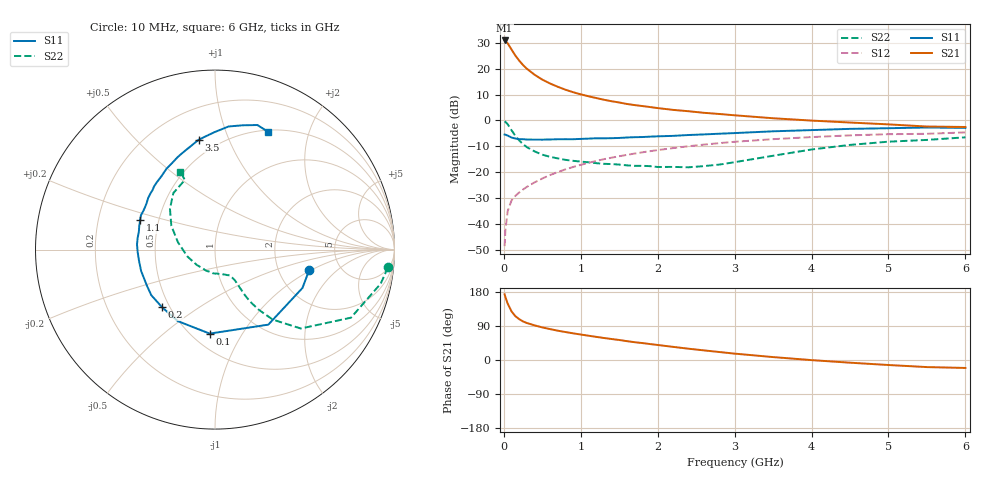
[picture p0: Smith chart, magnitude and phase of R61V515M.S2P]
! SIEMENS Small Signal Semiconductors
! BFR193
! Si NPN RF Bipolar Junction Transistor in SOT23
! VCE = 1.5 V  IC = 15 mA
! Common Emitter S-Parameters:  May  1996
# GHz  S  MA  R  50
!  f  S11  S21  S12  S22
! GHz  MAG  ANG  MAG  ANG  MAG  ANG  MAG  ANG
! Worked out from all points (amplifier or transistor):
!   36 points, 10 MHz to 6 GHz, reference 50 ohm
!   highest |S21| = 30.8 dB at 10 MHz (marker M1)
!   |S21| within 3 dB of that: start of sweep to 89.89 MHz
!   unconditionally stable (mu >= 1): 597.2 MHz to 1.991 GHz
!   at 250 MHz: K = 0.77, MSG = 24.0 dB, |S12| = -26.6 dB
!   at 1.4 GHz: K = 1.03, MAG = 9.7 dB, |S12| = -14.3 dB
!   at 6 GHz: K = 0.96, MSG = 1.0 dB, |S12| = -4.6 dB
!   S11 on the Smith chart (normalised r, x): 10 MHz: 2.98, -0.96; 100 MHz: 0.61, -0.73; 200 MHz: 0.45, -0.36; 1.1 GHz: 0.39, +0.16; 3.5 GHz: 0.39, +0.78; 6 GHz: 0.52, +1.41
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0.01  0.537 -12.3  34.79 173.2  0.0038 84.4  0.9685 -5.9
0.02  0.5321 -23.7  34.1 166.4  0.0077 80.9  0.9427 -11.6
0.05  0.5129 -54.6  30.59 148.8  0.018 69.9  0.8472 -26.6
0.1  0.469 -93.6  23.31 128.3  0.0289 61.3  0.6495 -42.6
0.15  0.4492 -117.6  17.77 115.6  0.0354 57.8  0.5052 -50.5
0.2  0.436 -132.7  14.2 107.7  0.0411 58.5  0.4136 -54.0
0.25  0.4365 -144.4  11.67 101.7  0.0469 59.3  0.349 -56.0
0.3  0.4292 -152.4  9.906 97.6  0.0528 60.9  0.3067 -56.7
0.4  0.4285 -163.9  7.602 91.4  0.0643 63.0  0.254 -56.9
0.5  0.4279 -171.7  6.131 86.0  0.0764 64.4  0.2198 -56.9
0.6  0.4311 -178.2  5.163 81.6  0.089 65.1  0.1996 -57.3
0.7  0.4355 176.2  4.466 77.4  0.1013 65.8  0.1864 -58.1
0.8  0.4359 171.3  3.923 73.8  0.1144 65.6  0.1748 -59.2
0.9  0.4355 167.0  3.508 70.4  0.1272 65.2  0.1672 -60.3
1.1  0.4481 158.7  2.93 64.1  0.153 64.1  0.1566 -64.9
1.3  0.4537 151.4  2.511 58.1  0.1797 62.2  0.1464 -70.3
1.6  0.4706 142.3  2.081 49.7  0.2178 59.1  0.1368 -81.6
2.2  0.5059 126.2  1.601 34.7  0.2941 51.3  0.1277 -111.9
3.5  0.6191 98.4  1.105 7.7  0.4372 31.5  0.2094 169.1
4.5  0.6901 83.7  0.914 -7.1  0.5172 16.9  0.3388 137.8
5.5  0.7332 71.2  0.765 -18.7  0.5545 2.5  0.4227 113.4
6  0.7202 65.9  0.75 -21.0  0.5901 -1.8  0.4744 114.0
